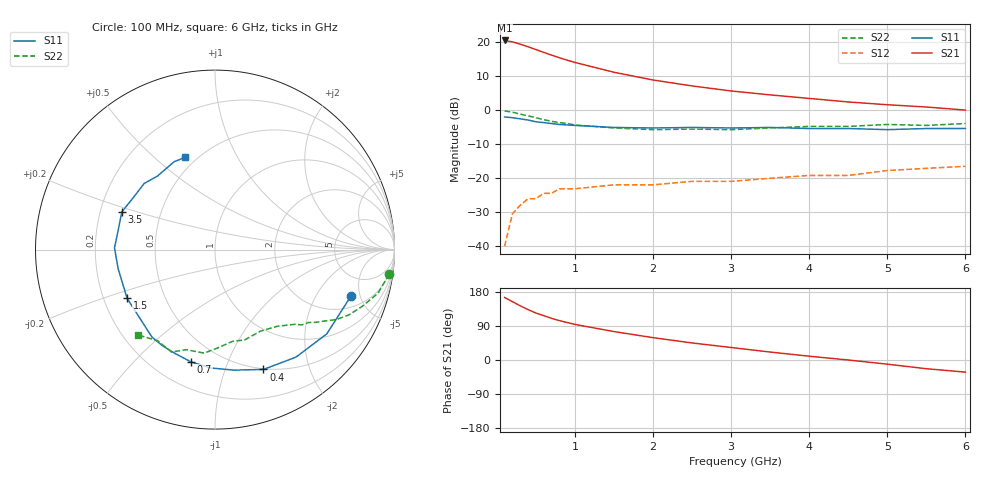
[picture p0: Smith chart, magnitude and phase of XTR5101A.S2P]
! HXTR-5101  (2N6701) Common Emitter
! Vce=18V  Ic=30mA
# ghz s ma r 50
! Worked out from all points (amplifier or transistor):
!   20 points, 100 MHz to 6 GHz, reference 50 ohm
!   highest |S21| = 20.6 dB at 100 MHz (marker M1)
!   |S21| within 3 dB of that: start of sweep to 539.8 MHz
!   unconditionally stable (mu >= 1): 1.896 GHz to end of sweep
!   at 400 MHz: K = 0.29, MSG = 22.4 dB, |S12| = -26.0 dB
!   at 1.5 GHz: K = 0.80, MSG = 16.6 dB, |S12| = -21.9 dB
!   at 6 GHz: K = 1.11, MAG = 6.3 dB, |S12| = -16.5 dB
!   S11 on the Smith chart (normalised r, x): 100 MHz: 2.83, -4.10; 400 MHz: 0.49, -1.36; 700 MHz: 0.35, -0.75; 1.5 GHz: 0.30, -0.24; 3.5 GHz: 0.29, +0.18; 6 GHz: 0.44, +0.63
0.1  0.8 -19.0  10.7 165.0  0.01 77.0  0.98 -8.0
0.2  0.78 -37.0  10.2 154.0  0.03 67.0  0.94 -15.0
0.3  0.75 -53.0  9.44 143.0  0.04 60.0  0.88 -21.0
0.4  0.72 -68.0  8.63 133.0  0.05 53.0  0.83 -26.0
0.5  0.68 -81.0  7.87 124.0  0.05 47.0  0.78 -30.0
0.6  0.66 -92.0  7.15 117.0  0.06 42.0  0.73 -33.0
0.7  0.64 -102.0  6.52 110.0  0.06 39.0  0.69 -36.0
0.8  0.62 -111.0  5.96 104.0  0.07 36.0  0.66 -38.0
0.9  0.61 -119.0  5.49 99.0  0.07 33.0  0.64 -41.0
1  0.6 -126.0  5.08 94.0  0.07 31.0  0.61 -43.0
1.5  0.56 -151.0  3.64 75.0  0.08 25.0  0.55 -51.0
2  0.55 -169.0  2.8 59.0  0.08 22.0  0.52 -61.0
2.5  0.56 179.0  2.29 45.0  0.09 21.0  0.53 -72.0
3  0.55 168.0  1.93 33.0  0.09 21.0  0.52 -79.0
3.5  0.56 158.0  1.69 21.0  0.1 20.0  0.55 -89.0
4  0.54 148.0  1.5 10.0  0.11 19.0  0.58 -96.0
4.5  0.54 137.0  1.33 0.0  0.11 18.0  0.58 -106.0
5  0.52 128.0  1.21 -11.0  0.13 16.0  0.62 -113.0
5.5  0.54 115.0  1.12 -23.0  0.14 14.0  0.6 -122.0
6  0.54 108.0  1.01 -32.0  0.15 11.0  0.64 -132.0
